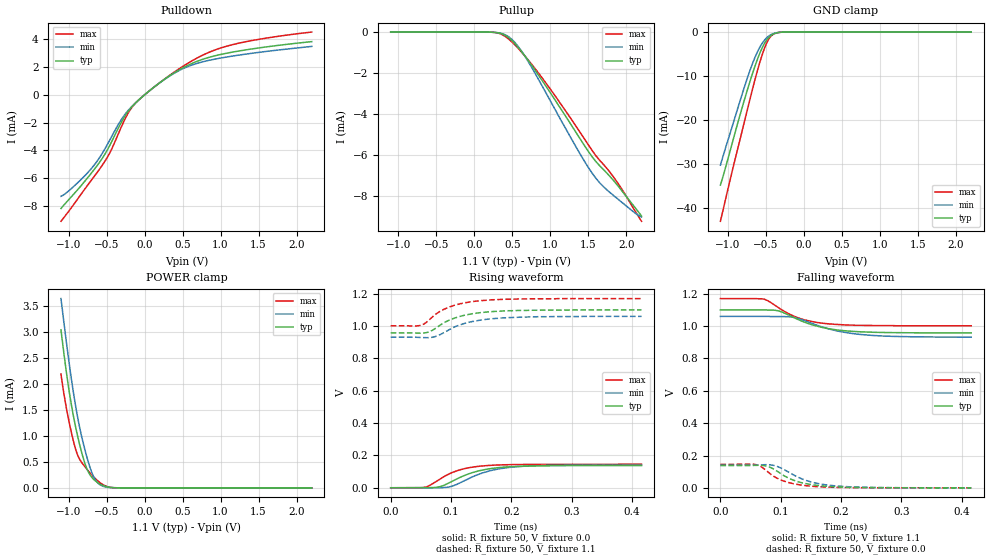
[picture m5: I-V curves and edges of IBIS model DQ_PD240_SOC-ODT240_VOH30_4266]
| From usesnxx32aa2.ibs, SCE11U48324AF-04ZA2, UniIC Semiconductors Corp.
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| DQ_PD240_SOC-ODT240_VOH30_4266
| (240 Ohm Pulldown, 240 Ohm System ODT Setting, VOH=VDDQ/3.0, 3200-4266Mbps)
[Model]   DQ_PD240_SOC-ODT240_VOH30_4266
Model_type   I/O
Vinl = 123.333mV
Vinh = 243.333mV
Vmeas = 183.333mV
Vref = 0.0mV
Cref = 0.0pF
Rref = 240.000Ohm
|   typ   min   max
|C_comp   0.797pF   0.747pF   0.847pF
C_comp_pullup   0.3985pF   0.3735pF   0.4235pF
C_comp_pulldown   0.3985pF   0.3735pF   0.4235pF
| Note: C_comp changes when the ODT circuit is enabled.
[Model Spec]
| Input threshold voltage corners
Vinl   0.1233V   0.1167V   0.1350V
Vinh   0.2433V   0.2367V   0.2550V
| Measurement voltage corners
Vmeas   0.1833V   0.1767V   0.1950V
| Timing spec test load voltage corners
Vref   0.0000V   0.0000V   0.0000V
| Dynamic Overshoot Parameters from LPDDR4 Specification
D_overshoot_ampl_h   0.30   NA   NA
D_overshoot_ampl_l   0.30   NA   NA
D_overshoot_area_h   0.1n   NA   NA
D_overshoot_area_l   0.1n   NA   NA
[Receiver Thresholds]
Vth   = 0.1833V
Vth_min  = 0.1800V
Vth_max  = 0.1866V
Vinh_ac  = 0.060V
Vinh_dc  = 0.060V
Vinl_ac  = -0.060V
Vinl_dc  = -0.060V
Tslew_ac = 5.000ns |Not specified, so set to high value
Threshold_sensitivity = 0.1667
Reference_supply Pullup_ref
[Voltage Range]   1.1000V   1.0600V   1.1700V
[Pullup Reference]   1.1000V   1.0600V   1.1700V
| Junction Temperature (Ambient temp is 35C typ 95C min -40C max)
[Temperature Range]   50.0   110.0   -40.0
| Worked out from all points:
|   slope of the pulldown table from 0 to 0.165 V, typ, clamps not added: 227 ohm
|   slope of the pullup table from 0 to 0.165 V, typ, clamps not added: 80.7 kohm
|   GND clamp passes 1 mA (typ) near -0.45 V on its own axis
|   POWER clamp passes 1 mA (typ) near -0.88 V on its own axis
|   rising waveform, R_fixture 50, V_fixture 0.0: 20-80 % time 57ps typ, 59.3ps min, 48.8ps max; typ from 0 V to 0.137 V
|   falling waveform, R_fixture 50, V_fixture 1.1: 20-80 % time 64.7ps typ, 73ps min, 56.1ps max; typ from 1.1 V to 0.958 V
|   rising waveform, R_fixture 50, V_fixture 1.1: 20-80 % time 54.2ps typ, 57.5ps min, 50.2ps max; typ from 0.958 V to 1.1 V
|   falling waveform, R_fixture 50, V_fixture 0.0: 20-80 % time 48.5ps typ, 53.9ps min, 43.9ps max; typ from 0.137 V to 0 V
[Pulldown]
|   Voltage   I(typ)   I(min)   I(max)
-1.1V     -8.17mA    -7.293mA   -9.087mA
-869mV    -6.746mA   -6.261mA   -7.4mA
-664.4mV  -5.376mA   -5.058mA   -5.876mA
-469.7mV  -3.757mA   -3.371mA   -4.293mA
-308mV    -2.001mA   -1.801mA   -2.335mA
-176mV    -919.6uA   -889.4uA   -974.2uA
-50.6mV   -245.1uA   -243.6uA   -239.1uA
246.4mV   1.053mA    1.042mA    1.061mA
569.8mV   2.115mA    2.026mA    2.264mA
979mV     2.868mA    2.616mA    3.32mA
1.484V    3.349mA    3.032mA    3.965mA
2.2V      3.818mA    3.475mA    4.505mA
[GND Clamp]
|   Voltage   I(typ)   I(min)   I(max)
-1.1V     -34.88mA   -30.34mA   -43.13mA
-1.047V   -31.79mA   -27.25mA   -39.23mA
-938.3mV  -24.92mA   -21.15mA   -31.24mA
-796.4mV  -16.18mA   -13.19mA   -21.29mA
-667.7mV  -8.939mA   -6.742mA   -12.34mA
-591.8mV  -5.271mA   -3.798mA   -7.523mA
-522.5mV  -2.673mA   -1.905mA   -3.822mA
-469.7mV  -1.361mA   -986.7uA   -1.791mA
-416.9mV  -601.5uA   -440.8uA   -665.5uA
-350.9mV  -167.8uA   -126.1uA   -148.2uA
-248.6mV  -12.24uA   -10.96uA   -7.123uA
2.2V      0A         0A         0A
[Pullup]
|   Voltage   I(typ)   I(min)   I(max)
-1.1V     1.047uA    1.615uA    471.8nA
239.8mV   -9.287uA   -9.208uA   -9.959uA
348.7mV   -70.57uA   -57.98uA   -97.34uA
457.6mV   -294.6uA   -245.6uA   -360.3uA
569.8mV   -714uA     -668.3uA   -763.6uA
688.6mV   -1.278mA   -1.312mA   -1.267mA
1.065V    -3.325mA   -3.788mA   -3.117mA
1.398V    -5.241mA   -5.982mA   -4.926mA
1.563V    -6.142mA   -6.945mA   -5.84mA
1.698V    -6.702mA   -7.534mA   -6.451mA
1.887V    -7.482mA   -8.134mA   -7.355mA
2.2V      -8.971mA   -9.017mA   -9.226mA
[POWER Clamp]
|   Voltage   I(typ)   I(min)   I(max)
-1.1V     3.036mA    3.636mA    2.186mA
-1.044V   2.383mA    2.969mA    1.654mA
-984.5mV  1.784mA    2.311mA    1.206mA
-911.9mV  1.201mA    1.611mA    764.9uA
-855.8mV  838uA      1.172mA    552.1uA
-783.2mV  462.1uA    720.1uA    402.5uA
-710.6mV  232.2uA    359.1uA    273.1uA
-657.8mV  146.8uA    178.8uA    190.7uA
-595.1mV  80.78uA    68.31uA    109.2uA
-482.9mV  15.79uA    9.506uA    19.51uA
-360.8mV  1.019uA    775nA      799.8nA
2.2V      0A         0A         0A
[Ramp]
|   typ   min   max
| 20% - 80%
dV/dt_r   82.35m/57.02p   84.10m/59.28p   87.12m/48.77p
dV/dt_f   85.23m/64.66p   76.87m/73.20p   100.80m/55.66p
| 25% - 75%
|dV/dt_r   68.62m/45.44p   70.08m/47.22p   72.60m/38.73p
|dV/dt_f   71.02m/51.53p   64.06m/58.26p   84.00m/44.10p
R_load = 50
[Rising Waveform]
R_fixture = 50
V_fixture = 0.0
|   Time   V(typ)   V(min)   V(max)
0s        184.7uV    156.9uV    135.9uV
57ps      -128.4uV   -56.27uV   3.425mV
78ps      3.819mV    135.6uV    45.42mV
95ps      26.93mV    3.878mV    82.36mV
106ps     47.95mV    15.54mV    100.1mV
120ps     72.52mV    39.85mV    116.2mV
154ps     111.2mV    93.93mV    135.8mV
188ps     127.8mV    121.9mV    142.3mV
225ps     134.3mV    134.1mV    144.4mV
416ps     137.4mV    140.3mV    145.3mV
[Falling Waveform]
R_fixture   = 50
V_fixture   = 1.1
V_fixture_min = 1.06
V_fixture_max = 1.17
|   Time   V(typ)   V(min)   V(max)
0s        1.1V       1.06V      1.17V
72ps      1.1V       1.06V      1.167V
94ps      1.096V     1.059V     1.12V
106ps     1.08V      1.059V     1.091V
126ps     1.046V     1.05V      1.055V
151ps     1.009V     1.018V     1.029V
173ps     988.4mV    989.9mV    1.016V
208ps     970.7mV    960mV      1.007V
253ps     961.9mV    942.1mV    1.003V
416ps     958mV      931.9mV    1.002V
[Rising Waveform]
R_fixture   = 50
V_fixture   = 1.1
V_fixture_min = 1.06
V_fixture_max = 1.17
|   Time   V(typ)   V(min)   V(max)
0s        957.9mV    931.6mV    1.002V
50ps      955.9mV    929.5mV    1.005V
58ps      958.6mV    928.3mV    1.02V
72ps      980.5mV    933.2mV    1.066V
92ps      1.028V     967.8mV    1.11V
114ps     1.059V     1.007V     1.137V
140ps     1.079V     1.031V     1.154V
172ps     1.091V     1.047V     1.163V
219ps     1.097V     1.056V     1.168V
416ps     1.1V       1.06V      1.17V
[Falling Waveform]
R_fixture = 50
V_fixture = 0.0
|   Time   V(typ)   V(min)   V(max)
0s        137.5mV    140.4mV    145.4mV
58ps      139.5mV    141.4mV    144.5mV
69ps      139mV      143.4mV    127.2mV
86ps      120.8mV    140.6mV    77.13mV
99ps      90.77mV    125.2mV    51.02mV
116ps     55.15mV    91.02mV    30mV
147ps     22.34mV    40.06mV    11.43mV
177ps     9.473mV    17.66mV    4.55mV
219ps     2.994mV    5.766mV    1.384mV
416ps     270uV      288.1uV    171.4uV
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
